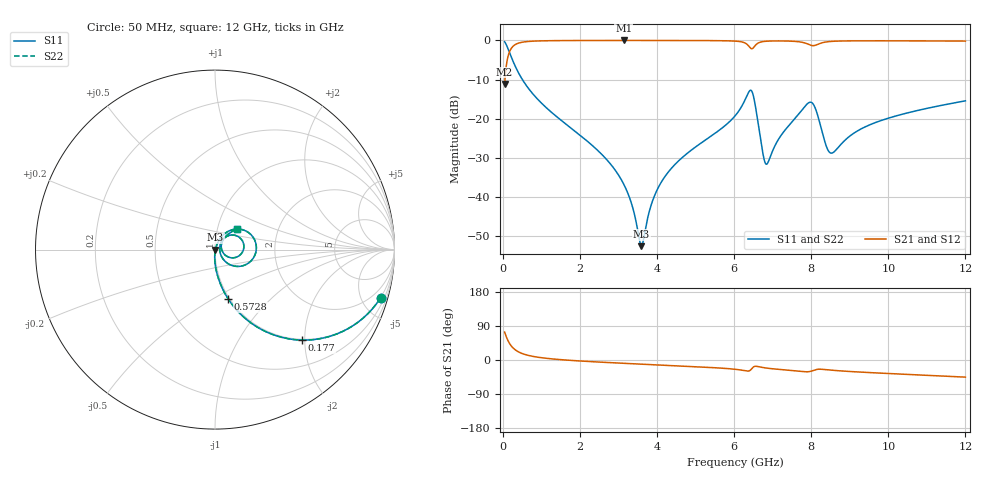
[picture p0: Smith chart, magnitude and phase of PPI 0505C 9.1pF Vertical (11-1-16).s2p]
# GHz S MA R 50
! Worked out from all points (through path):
!   1601 points, 50 MHz to 12 GHz, reference 50 ohm
!   highest |S21| = -0.02 dB at 3.142 GHz (marker M1); lowest = -11.2 dB at 50 MHz (marker M2)
!   group delay of S21, straight-line fit = 13.5 ps
!   lowest |S11| = -52.6 dB at 3.598 GHz (marker M3), VSWR 1.00, Z = 50.2 - j0.05 ohm
!   |S11| at or under -10 dB: 510.5 MHz to end of sweep
!   |S22| runs from -52.6 to -0.3 dB; largest |S21 - S12| = 0
!   S11 on the Smith chart (normalised r, x): 50 MHz: 0.98, -6.87; 177 MHz: 0.98, -1.94; 572.8 MHz: 0.98, -0.59; 12 GHz: 1.24, +0.29
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0.05  0.9608 -16.2  0.277 73.8  0.277 73.8  0.9608 -16.2
0.1769688  0.699 -46.2  0.7147 43.8  0.7147 43.8  0.699 -46.2
0.3338125  0.458 -63.7  0.8882 26.2  0.8882 26.2  0.458 -63.7
0.5728125  0.2835 -75.1  0.958 14.7  0.958 14.7  0.2835 -75.1
2.044156  0.0594 -91.2  0.9964 -2.8  0.9964 -2.8  0.0594 -91.2
3.142063  0.0145 -90.2  0.9975 -8.8  0.9975 -8.8  0.0145 -90.2
3.351187  0.00795 -83.4  0.9975 -9.8  0.9975 -9.8  0.00795 -83.4
3.597656  0.002357 -12.2  0.9974 -11.0  0.9974 -11.0  0.002357 -12.2
3.844125  0.007716 59.1  0.9972 -12.1  0.9972 -12.1  0.007716 59.1
4.038312  0.01329 65.7  0.9971 -13.0  0.9971 -13.0  0.01329 65.7
4.583531  0.02961 68.6  0.9963 -15.6  0.9963 -15.6  0.02961 68.6
6.025  0.1085 57.7  0.9789 -24.4  0.9789 -24.4  0.1085 57.7
6.316281  0.1876 36.5  0.9068 -28.9  0.9068 -28.9  0.1876 36.5
6.458188  0.2255 -6.8  0.7812 -23.2  0.7812 -23.2  0.2255 -6.8
6.756938  0.03418 -32.2  0.9661 -20.0  0.9661 -20.0  0.03418 -32.2
6.846563  0.02627 5.5  0.9761 -21.4  0.9761 -21.4  0.02627 5.5
7.27975  0.06722 51.8  0.9828 -25.7  0.9828 -25.7  0.06722 51.8
8.019156  0.1601 2.3  0.859 -28.9  0.859 -28.9  0.1601 2.3
8.519562  0.03632 9.0  0.9698 -26.8  0.9698 -26.8  0.03632 9.0
9.184281  0.06901 49.9  0.9867 -31.4  0.9867 -31.4  0.06901 49.9
10.01331  0.102 50.3  0.9871 -35.7  0.9871 -35.7  0.102 50.3
12  0.169 42.8  0.9789 -45.2  0.9789 -45.2  0.169 42.8
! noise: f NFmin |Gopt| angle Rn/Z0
0.05  0.0004776  0.8924  1.496  0.0009674
1.372  0.004497  0.7058  4.582  0.002997
2.701  0.007421  0.6591  8.398  0.004137
4.031  0.01035  0.6406  12.2  0.005381
5.36  0.01566  0.6785  16.01  0.009239
6.682  0.05857  0.8806  20.2  0.1029
8.012  0.11  0.9226  24.07  0.3009
9.341  0.02939  0.703  27.67  0.01833
10.67  0.02607  0.6361  30.98  0.01258
12  0.02704  0.6145  34.27  0.01197
